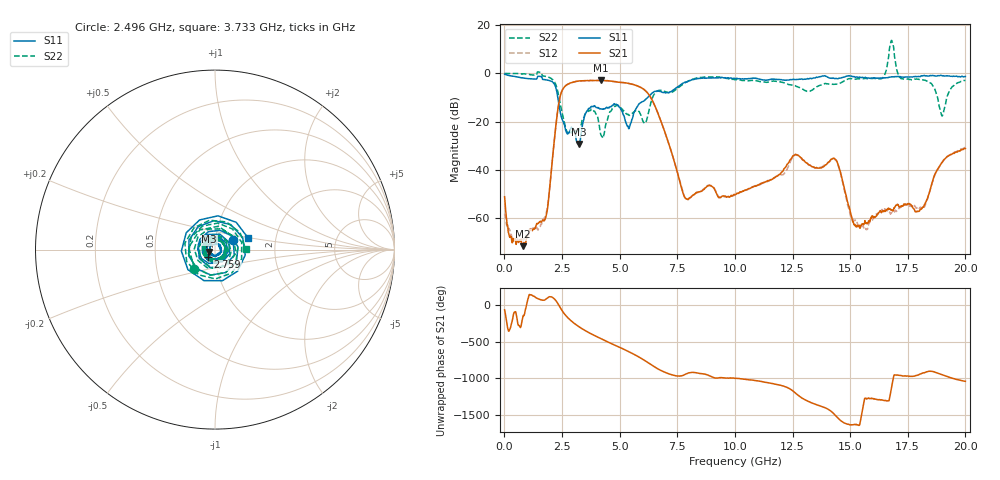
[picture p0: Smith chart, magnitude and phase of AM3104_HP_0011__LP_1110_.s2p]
!Created with skrf (http://scikit-rf.org).
# Hz S RI R 50.0
!freq ReS11 ImS11 ReS21 ImS21 ReS12 ImS12 ReS22 ImS22
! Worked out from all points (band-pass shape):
!   1601 points, 10 MHz to 20 GHz, reference 50 ohm
!   highest |S21| = -2.89 dB at 4.183 GHz (marker M1); lowest = -71.6 dB at 809.6 MHz (marker M2)
!   |S21| within 3 dB of the highest: 2.583 GHz to 5.924 GHz (3.341 GHz wide, 78.5 % of centre)
!   lowest |S11| = -29.3 dB at 3.221 GHz (marker M3), VSWR 1.07, Z = 46.8 - j1.07 ohm
!   |S11| at or under -10 dB: 2.318 GHz to 6.216 GHz (3.899 GHz wide, 91.4 % of centre)
!   |S22| runs from -26.8 to 13.6 dB; largest |S21 - S12| = 0.077
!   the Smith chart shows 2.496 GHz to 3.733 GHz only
!   S11 on the Smith chart (normalised r, x): 2.496 GHz: 1.22, +0.14; 2.759 GHz: 0.92, -0.08; 3.733 GHz: 1.44, +0.19
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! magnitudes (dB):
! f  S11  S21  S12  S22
! 10 MHz  -0.3  -51.1  -58.2  -0.1
! 259.9 MHz  -1.0  -67.6  -66.5  -0.1
! 809.6 MHz  -1.9  -71.6  -69.0  -0.2
! 1.797 GHz  -2.7  -59.6  -58.7  -1.3
! 2.496 GHz  -18.8  -7.3  -7.3  -16.1
! 2.759 GHz  -24.9  -4.5  -4.5  -24.6
! 3.221 GHz  -29.3  -3.2  -3.3  -24.3
! 3.346 GHz  -23.7  -3.1  -3.2  -20.9
! 3.733 GHz  -14.2  -3.0  -3.0  -15.3
! 4.183 GHz  -14.8  -2.9  -2.9  -25.4
! 5.395 GHz  -22.9  -4.2  -4.2  -17.4
! 6.107 GHz  -11.0  -7.1  -7.1  -20.6
! 6.682 GHz  -7.3  -17.0  -17.1  -7.1
! 7.869 GHz  -3.6  -51.8  -51.9  -3.7
! 10.01 GHz  -2.2  -50.4  -50.4  -2.7
! 13.34 GHz  -2.2  -38.6  -38.7  -7.0
! 14.37 GHz  -2.1  -35.8  -36.0  -4.5
! 15.25 GHz  -1.6  -63.3  -61.1  -2.4
! 16.68 GHz  -1.6  -56.0  -57.5  7.3
! 18.04 GHz  -1.4  -56.4  -55.5  -2.6
! 18.99 GHz  -1.1  -37.0  -36.8  -17.7
! 20 GHz  -1.3  -31.2  -30.8  -2.9
